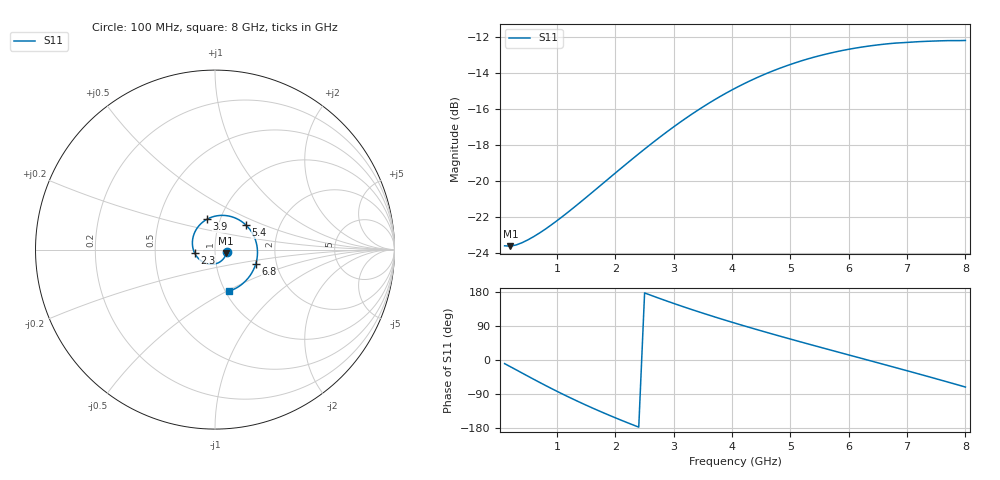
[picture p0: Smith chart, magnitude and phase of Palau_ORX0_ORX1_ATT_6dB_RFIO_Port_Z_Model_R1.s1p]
! Created Fri Oct  9 14:29:16 2020
! Palau ORX0/ORX1 RFIO Port Impedance Model.
! Attenuation  : 6 dB.
! Revision		: R1.
! Impedance Mode 	: Balanced Differential-Mode.
! Impedance Format 	: Series Equivalent Differential Impedance (SEDZ).
# hz S ma R 100
! 1 Port Network Data from SP1.SP block
! freq  magS11  angS11
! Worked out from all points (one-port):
!   80 points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, 100 MHz to 8 GHz, reference 100 ohm
!   lowest |S11| = -23.6 dB at 200 MHz (marker M1), VSWR 1.14, Z = 113 - j4.6 ohm
!   |S11| at or under -10 dB: start of sweep to end of sweep
!   S11 on the Smith chart (normalised r, x): 100 MHz: 1.14, -0.03; 2.3 GHz: 0.79, -0.03; 3.9 GHz: 0.87, +0.30; 5.4 GHz: 1.35, +0.39; 6.8 GHz: 1.56, -0.27; 8 GHz: 1.04, -0.51
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1e8  0.06622 -9.6
2e8  0.06606 -17.8
4e8  0.06755 -34.4
6e8  0.07024 -51.0
1.1e9  0.07999 -90.4
1.4e9  0.08746 -112.3
1.6e9  0.09301 -126.3
1.8e9  0.09898 -139.7
2.1e9  0.1086 -158.9
2.3e9  0.1155 -171.2
2.7e9  0.13 165.6
3.1e9  0.1452 143.9
3.5e9  0.1605 123.6
3.9e9  0.1753 104.3
4.1e9  0.1824 95.0
4.4e9  0.1925 81.4
4.6e9  0.1989 72.5
4.8e9  0.2048 63.8
5.1e9  0.213 51.0
5.4e9  0.2202 38.3
5.8e9  0.2283 21.7
6.1e9  0.2332 9.2
6.5e9  0.2383 -7.4
6.8e9  0.241 -20.0
7.1e9  0.2427 -32.6
7.3e9  0.2436 -41.0
7.6e9  0.2446 -53.9
8e9  0.2451 -71.3
